FUNCTION_BLOCK FB_PushPopCutter
VAR_IN_OUT
	ArrayCutterEnc: ARRAY[1..INUM] OF LREAL;
END_VAR
VAR_INPUT
	PushCutterEnc:  LREAL;
END_VAR
VAR_OUTPUT
	PopCutterEnc	: LREAL;
	busy						: BOOL;
END_VAR
VAR
	i: INT;
END_VAR

;

METHOD PopStack : BOOL
VAR_INPUT
END_VAR

VAR
	i: INT;
END_VAR
busy:=TRUE;
PopCutterEnc:=ArrayCutterEnc[1];
FOR i:=2 TO INUM DO
	ArrayCutterEnc[i-1]:=ArrayCutterEnc[i];
END_FOR
ArrayCutterEnc[INUM]	:=	0;
busy:=FALSE;
END_METHOD

METHOD PushStack : BOOL
VAR_INPUT
END_VAR
busy:=TRUE;
FOR i:=1 TO INUM DO
	IF  ArrayCutterEnc[i]=0 THEN
		ArrayCutterEnc[i]:=PushCutterEnc;
		EXIT;
	END_IF
END_FOR
busy:=FALSE;
END_METHOD

END_FUNCTION_BLOCK
